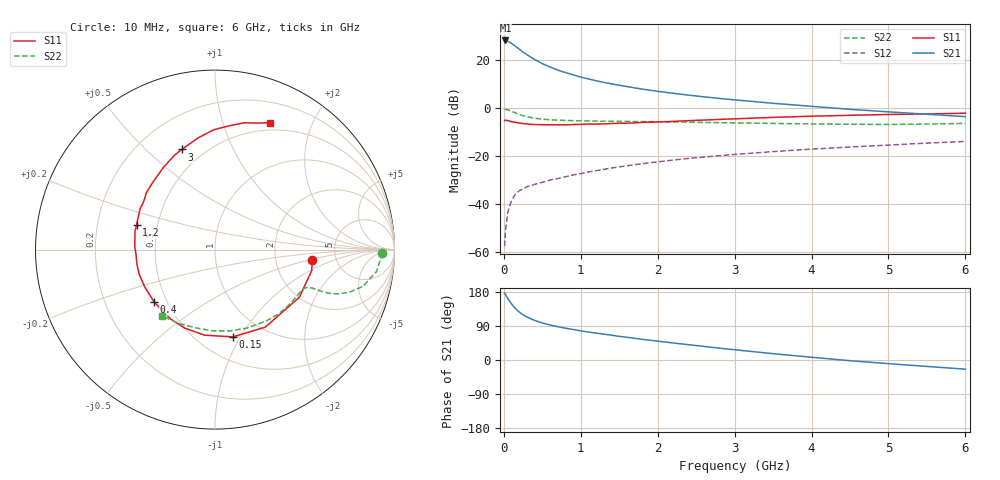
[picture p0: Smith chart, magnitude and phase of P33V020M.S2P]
! SIEMENS Small Signal Semiconductors
! BFP181
! Si NPN RF Bipolar Junction Transistor in SOT143
! VCE = 3 V  IC = 20 mA
! Common Emitter S-Parameters:  March  1996
# GHz  S  MA  R  50
!  f  S11  S21  S12  S22
! GHz  MAG  ANG  MAG  ANG  MAG  ANG  MAG  ANG
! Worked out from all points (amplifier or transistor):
!   36 points, 10 MHz to 6 GHz, reference 50 ohm
!   highest |S21| = 28.1 dB at 20 MHz (marker M1)
!   |S21| within 3 dB of that: start of sweep to 175.3 MHz
!   unconditionally stable (mu >= 1): start of sweep to 16.09 MHz; 461.3 MHz to end of sweep
!   at 250 MHz: K = 0.67, MSG = 28.5 dB, |S12| = -33.8 dB
!   at 1.4 GHz: K = 1.46, MAG = 13.5 dB, |S12| = -25.1 dB
!   at 6 GHz: K = 1.11, MAG = 3.2 dB, |S12| = -14.0 dB
!   S11 on the Smith chart (normalised r, x): 10 MHz: 3.30, -0.54; 150 MHz: 0.72, -0.93; 400 MHz: 0.43, -0.31; 1.2 GHz: 0.38, +0.13; 3 GHz: 0.38, +0.65; 6 GHz: 0.41, +1.44
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0.01  0.5448 -6.1  25.36 176.4  0.0013 78.8  0.9287 -1.1
0.02  0.5514 -12.3  25.37 173.3  0.0026 78.2  0.9252 -2.9
0.05  0.5399 -29.4  24.57 163.0  0.0065 78.6  0.9084 -7.7
0.1  0.5149 -57.1  21.95 148.1  0.0117 66.4  0.8499 -13.9
0.15  0.4964 -78.5  19.28 136.0  0.0157 60.0  0.7839 -17.7
0.2  0.4801 -97.0  16.75 126.6  0.0186 56.9  0.7285 -19.8
0.25  0.469 -111.0  14.51 119.2  0.0204 53.0  0.6831 -20.9
0.3  0.4591 -122.3  12.79 113.6  0.0226 52.3  0.6495 -21.3
0.4  0.4474 -139.3  10.19 104.4  0.0253 52.3  0.606 -21.5
0.5  0.4435 -152.0  8.329 97.7  0.0279 51.8  0.5794 -21.6
0.6  0.4441 -162.1  7.115 92.5  0.0311 53.4  0.563 -22.0
0.7  0.4427 -169.5  6.124 88.0  0.0334 54.3  0.5519 -22.5
0.9  0.4474 177.7  4.867 80.5  0.0397 55.4  0.5394 -24.0
1.1  0.4577 167.2  3.995 73.7  0.0459 56.3  0.5312 -26.2
1.2  0.4573 162.8  3.666 71.0  0.0488 56.5  0.5284 -27.4
1.7  0.4844 143.8  2.603 57.2  0.0652 56.2  0.5176 -34.5
2.2  0.5202 128.4  2.008 44.9  0.0812 54.0  0.5064 -42.6
3  0.588 108.4  1.464 27.1  0.1065 48.8  0.4835 -57.4
3.5  0.6303 98.4  1.241 16.7  0.1219 45.4  0.4719 -67.9
4.5  0.6964 83.0  0.929 -1.9  0.1521 37.3  0.453 -91.6
5.5  0.7426 71.7  0.733 -17.0  0.1835 29.3  0.4583 -116.2
6  0.7706 66.5  0.654 -24.2  0.1985 24.7  0.473 -128.4
